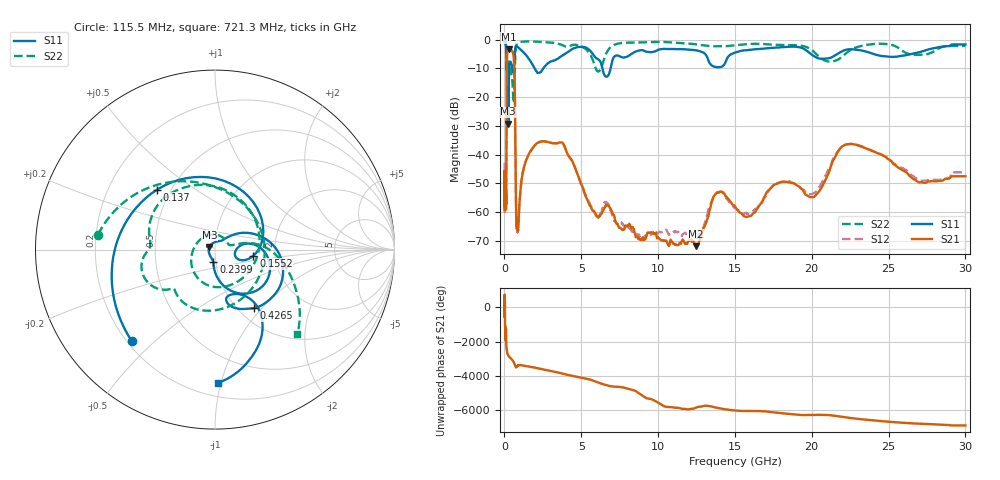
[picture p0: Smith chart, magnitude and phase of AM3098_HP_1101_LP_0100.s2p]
! Date/Time: Thu, Feb 28, 2019 8:45 AM
! Network Analyzer: Agilent Technologies E8364B Rev: A.07.50.67
! Sweep from 0.010 to 30.000 GHz, 1601 Points, Sweep Type: LOG
! Power Supply: 5.022 V, 0.002 A
# Hz S DB R 50
!freq MagS11 AngS11 MagS21 AngS21 MagS12 AngS12 MagS22 AngS22
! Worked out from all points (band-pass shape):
!   1601 points, 10 MHz to 30 GHz, reference 50 ohm
!   highest |S21| = -3.38 dB at 266.5 MHz (marker M1); lowest = -71.8 dB at 12.43 GHz (marker M2)
!   |S21| within 3 dB of the highest: 158.5 MHz to 606.5 MHz (448 MHz wide, 117 % of centre)
!   lowest |S11| = -29.3 dB at 250.9 MHz (marker M3), VSWR 1.07, Z = 47 + j1.45 ohm
!   |S11| at or under -10 dB: 207.3 MHz to 304.4 MHz (97.12 MHz wide, 38 % of centre); 1.96 GHz to 2.529 GHz (569.6 MHz wide, 25.4 % of centre); 6.371 GHz to 6.908 GHz (536.9 MHz wide, 8.09 % of centre)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
!   |S22| runs from -22.0 to -0.5 dB; largest |S21 - S12| = 0.012
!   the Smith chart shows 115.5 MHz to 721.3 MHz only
!   S11 on the Smith chart (normalised r, x): 115.5 MHz: 0.22, -0.42; 137 MHz: 0.42, +0.36; 155.2 MHz: 1.54, -0.11; 239.9 MHz: 0.97, -0.13; 426.5 MHz: 1.17, -0.90; 721.3 MHz: 0.30, -0.98
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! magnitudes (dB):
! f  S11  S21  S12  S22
! 10 MHz  -0.4  -46.0  -43.3  -0.5
! 38.04 MHz  -0.3  -57.9  -58.1  -0.7
! 115.5 MHz  -3.2  -55.8  -54.9  -3.6
! 137 MHz  -6.7  -24.7  -24.6  -10.8
! 144.7 MHz  -8.7  -14.2  -14.2  -10.3
! 155.2 MHz  -13.3  -7.3  -7.3  -9.4
! 206.4 MHz  -9.9  -4.0  -4.0  -7.5
! 239.9 MHz  -23.3  -3.5  -3.5  -8.7
! 250.9 MHz  -29.3  -3.4  -3.4  -8.8
! 266.5 MHz  -19.0  -3.4  -3.3  -8.8
! 426.5 MHz  -8.2  -3.6  -3.6  -11.4
! 550.5 MHz  -11.2  -4.6  -4.6  -18.8
! 652.6 MHz  -6.2  -11.4  -11.4  -13.8
! 721.3 MHz  -2.6  -42.9  -42.8  -3.6
! 769.7 MHz  -2.3  -63.1  -63.6  -1.9
! 842.3 MHz  -2.5  -65.3  -66.4  -1.2
! 2.084 GHz  -11.1  -36.2  -36.2  -0.7
! 3.779 GHz  -5.5  -35.9  -36.0  -1.9
! 7.926 GHz  -6.1  -64.9  -65.6  -1.1
! 12.43 GHz  -3.7  -71.8  -70.1  -1.6
! 22.56 GHz  -3.4  -36.3  -36.2  -3.5
! 30 GHz  -1.7  -47.5  -46.2  -2.2
